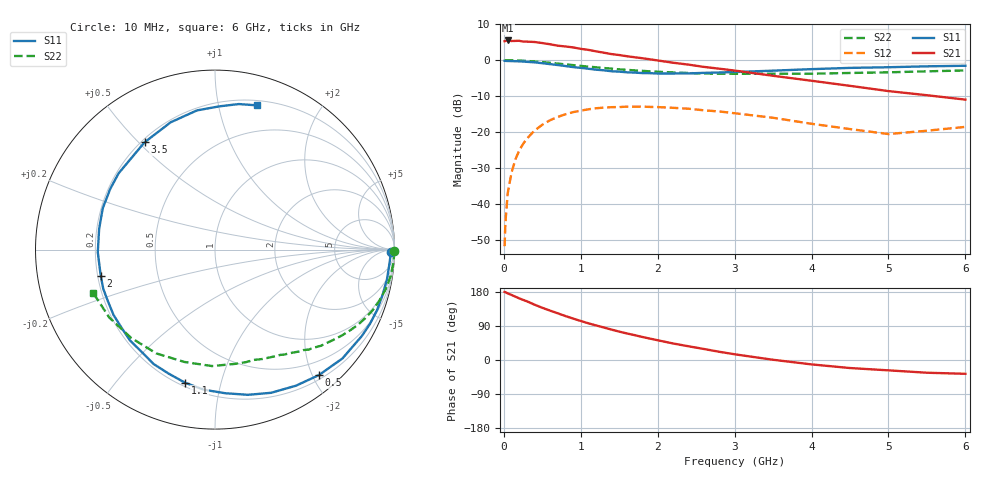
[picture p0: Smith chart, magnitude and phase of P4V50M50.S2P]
! SIEMENS Small Signal Semiconductors
! BFP182
! Si NPN RF Bipolar Junction Transistor in SOT143
! VCE = 0.5 V  IC = 0.5 mA
! Common Emitter S-Parameters:  March  1996
# GHz  S  MA  R  50
!  f  S11  S21  S12  S22
! GHz  MAG  ANG  MAG  ANG  MAG  ANG  MAG  ANG
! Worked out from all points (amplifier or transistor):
!   36 points, 10 MHz to 6 GHz, reference 50 ohm
!   highest |S21| = 5.5 dB at 50 MHz (marker M1)
!   |S21| within 3 dB of that: start of sweep to 1.191 GHz
!   unconditionally stable (mu >= 1): 2.65 GHz to end of sweep
!   at 250 MHz: K = 0.10, MSG = 14.2 dB, |S12| = -23.3 dB
!   at 1.4 GHz: K = 0.57, MSG = 7.4 dB, |S12| = -13.1 dB
!   at 6 GHz: K = 1.76, MAG = -1.3 dB, |S12| = -18.5 dB
!   S11 on the Smith chart (normalised r, x): 10 MHz: 62, -51; 500 MHz: 0.26, -2.10; 1.1 GHz: 0.22, -0.78; 2 GHz: 0.21, -0.11; 3.5 GHz: 0.21, +0.52; 6 GHz: 0.24, +1.31
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0.01  0.981 -0.9  1.837 179.6  0.0026 83.5  0.9985 -0.4
0.02  0.9785 -2.0  1.852 179.0  0.0054 88.2  0.9952 -0.8
0.05  0.9745 -5.2  1.881 175.8  0.0141 88.5  0.9981 -2.2
0.1  0.9725 -9.9  1.848 171.6  0.0274 82.4  0.9956 -4.4
0.15  0.9671 -15.4  1.856 167.2  0.0417 79.4  0.9928 -6.6
0.2  0.9638 -20.5  1.86 162.7  0.0556 76.6  0.989 -8.7
0.3  0.9492 -30.5  1.811 154.9  0.0814 69.4  0.9761 -13.1
0.4  0.9338 -40.5  1.791 145.9  0.1053 63.0  0.9603 -17.0
0.5  0.9076 -50.4  1.731 137.8  0.1268 56.5  0.9414 -21.0
0.8  0.8297 -77.2  1.553 116.0  0.1769 39.3  0.8745 -31.2
0.9  0.8021 -86.0  1.505 109.3  0.1897 34.4  0.8543 -34.0
1.1  0.7604 -102.6  1.391 96.7  0.2077 25.1  0.814 -39.5
1.5  0.6932 -133.1  1.18 74.9  0.2231 9.1  0.7453 -48.7
1.8  0.6625 -154.2  1.065 60.8  0.2262 0.2  0.7115 -54.3
2  0.6532 -167.1  0.991 52.1  0.223 -5.4  0.6908 -58.1
2.2  0.6532 -178.7  0.922 43.6  0.2177 -10.9  0.6763 -62.3
2.8  0.6745 150.0  0.762 21.7  0.1939 -23.4  0.6502 -74.7
3.5  0.7151 123.3  0.607 0.6  0.1584 -32.5  0.6491 -91.5
4.5  0.782 97.4  0.44 -21.2  0.1103 -30.4  0.6644 -119.5
5  0.7984 88.3  0.372 -27.3  0.0941 -18.9  0.6784 -133.5
5.5  0.8217 80.7  0.326 -33.6  0.1046 -7.4  0.7002 -147.3
6  0.8372 73.7  0.283 -36.4  0.1183 -2.5  0.7202 -160.3
